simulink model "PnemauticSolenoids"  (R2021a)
settings: Solver=VariableStepAuto  StartTime=0.0  StopTime=10.0  RelTol=1e-3
libraries: vexv5lib x6, vexcommonlib x1

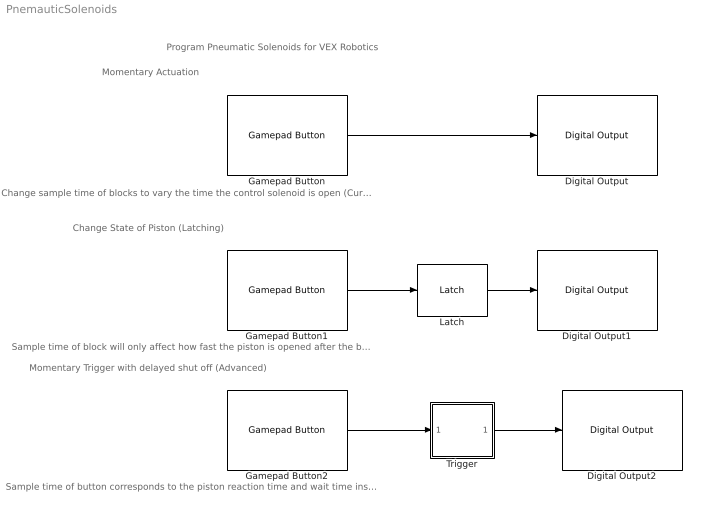
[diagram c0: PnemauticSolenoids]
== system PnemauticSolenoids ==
  note: Program Pneumatic Solenoids for VEX Robotics
  note: Change sample time of blocks to vary the time the control solenoid is open (Currently set to 0.5 seconds) Longer time intervals will affect reaction time
  note: Change State of Piston (Latching)
  note: Momentary Actuation
  note: Sample time of block will only affect how fast the piston is opened after the button is pressed
  note: Momentary Trigger with delayed shut off (Advanced)
  note: Sample time of button corresponds to the piston reaction time and wait time inside trigger chart corresponds to the time the solenoid is open.
  Digital Output : vexv5lib/Actuators/Digital Output  port=A
  Digital Output1 : vexv5lib/Actuators/Digital Output  port=A
  Digital Output2 : vexv5lib/Actuators/Digital Output  port=A
  Gamepad Button : vexv5lib/Gamepad/Gamepad Button  joystickType=Master  chan=R1  SampleTime=0.5
  Gamepad Button1 : vexv5lib/Gamepad/Gamepad Button  joystickType=Master  chan=R1  SampleTime=0.02
  Gamepad Button2 : vexv5lib/Gamepad/Gamepad Button  joystickType=Master  chan=R1  SampleTime=0.02
  Latch : vexcommonlib/Latch  output0=off  BlockPlatform=vexv5
  Trigger : Stateflow chart  TreatAsAtomicUnit=on
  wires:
  Gamepad Button/1 -> Digital Output/1
  Gamepad Button1/1 -> Latch/1
  Latch/1 -> Digital Output1/1
  Gamepad Button2/1 -> Trigger/1(input)
  Trigger/1(output) -> Digital Output2/1

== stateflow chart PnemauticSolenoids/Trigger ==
  state Idle
    output=0;
  state Wait
    output=1;
  (default) -> Idle : {output=0;}
  Idle -> Wait : [input]
  Wait -> Idle : after(0.5,sec)
  data: output output; input input
